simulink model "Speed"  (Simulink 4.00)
settings: Solver=ode45  StartTime=0.0  StopTime=1  MaxStep=0.0002  RelTol=1e-3
undefined symbols (not defined in the file or in its folder): const, J, No, Tf, Tmax, Ttc
libraries: simulink3 x2

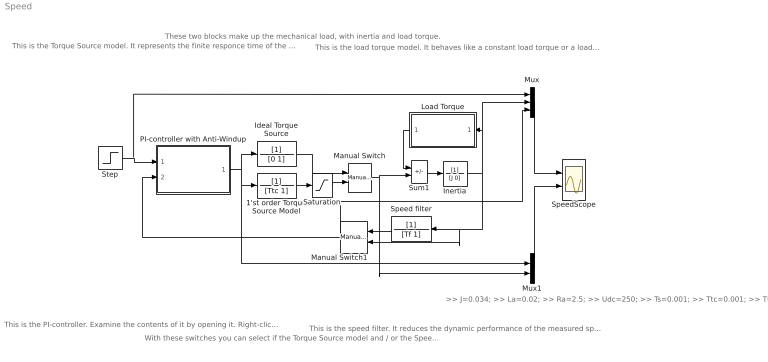
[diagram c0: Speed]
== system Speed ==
  note: This is the PI-controller. Examine the contents of it by opening it. Right-clic and select "Look under mask".
  note: With these switches you can select if the Torque Source model and / or the Speed Filter should be engaged.
  note: This is the load torque model. It behaves like a constant load torque or a load torque that is liearly or quadratically proportional to speed according to the user selection.
  note: These two blocks make up the mechanical load, with inertia and load torque.
  note: This is the Torque Source model. It represents the finite responce time of the torque loop as a 1'st order time constant and a limitation.
  note: This is the speed filter. It reduces the dynamic performance of the measured speed signal
  note: >> J=0.034; >> La=0.02; >> Ra=2.5; >> Udc=250; >> Ts=0.001; >> Ttc=0.001; >> Tf=0.05; >> Tmax=round(10*(16+rand*4))/10;
  1'st order Torque Source Model : TransferFcn  Numerator=[1]  Denominator=[Ttc 1]  AbsoluteTolerance=auto  Realization=auto
  Ideal Torque Source : TransferFcn  Numerator=[1]  Denominator=[0 1]  AbsoluteTolerance=auto  Realization=auto
  Inertia : TransferFcn  Numerator=[1]  Denominator=[J 0]  AbsoluteTolerance=auto  Realization=auto
  Load Torque : Subsystem  Orientation=left  mask(Speed dependent load){type=const, wn=100, Tn=0}
      mask prompts: type "Load type"; wn "Nominal speed [rad/s]"; Tn "Nominal load torque [Nm]"
      mask help: Either constant load torque, linearly dependent of speed or quadratically dependent of speed.
  Manual Switch : simulink3/Nonlinear/Manual Switch  sw=1  action=0
  Manual Switch1 : simulink3/Nonlinear/Manual Switch  Orientation=left  sw=0  action=0
  Mux : Mux  Inputs=3
  Mux1 : Mux  Inputs=2
  PI-controller with Anti-Windup : Subsystem  mask{Kp=0, Ti=inf, Ttc=Ttc, Limitoutput=No, Out_max=Tmax, Out_min=-Tmax}
      mask prompts: Kp "Gain"; Ti "Integral time constant"; Ttc "Controller Sampling Time"; Limitoutput "Limit the output"; Out_max "Max Controller Output (if limited)     INCLUDES Anti Windup !!"; Out_min "Min Controller Output (if limited)     INCLUDES Anti Windup !!"
  Saturation : Saturate  UpperLimit=Tmax  LowerLimit=-Tmax  LinearizeAsGain=on
  Speed filter : TransferFcn  Orientation=left  Numerator=[1]  Denominator=[Tf 1]  AbsoluteTolerance=auto  Realization=auto
  SpeedScope : Scope  NumInputPorts=2
  Step : Step  Time=0.2  Before=0  After=100  SampleTime=0
  Sum1 : Sum  Inputs=-+  SaturateOnIntegerOverflow=on
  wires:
  Inertia/1 -> Speed filter/1, Manual Switch1/2, Load Torque/1(w), Mux/2
  Mux/1 -> SpeedScope/1
  Sum1/1 -> Inertia/1
  Load Torque/1(Tl) -> Sum1/1
  Mux1/1 -> SpeedScope/2
  Step/1 -> PI-controller with Anti-Windup/1(Ref), Mux/1
  PI-controller with Anti-Windup/1(Out) -> 1'st order Torque Source Model/1, Mux1/1, Ideal Torque Source/1
  1'st order Torque Source Model/1 -> Saturation/1
  Manual Switch/1 -> Sum1/2, Mux1/2
  Speed filter/1 -> Manual Switch1/1
  Manual Switch1/1 -> PI-controller with Anti-Windup/2(Act), Mux/3
  Saturation/1 -> Manual Switch/2
  Ideal Torque Source/1 -> Manual Switch/1

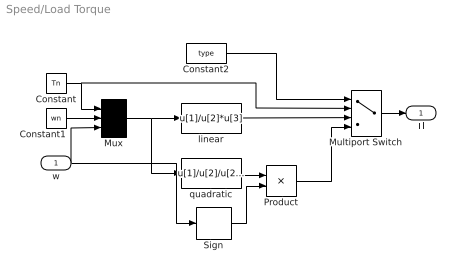
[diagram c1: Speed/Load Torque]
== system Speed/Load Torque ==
  w : Inport  Port=1  LatchInput=off
  Constant : Constant  Value=Tn
  Constant1 : Constant  Value=wn
  Constant2 : Constant  Value=type
  Multiport Switch : MultiPortSwitch  Inputs=3
  Mux : Mux  Inputs=3
  Product : Product  Inputs=2  Multiplication=Element-wise(.*)  SaturateOnIntegerOverflow=on
  Sign : Signum
  linear : Fcn  Expr=u[1]/u[2]*u[3]
  quadratic : Fcn  Expr=u[1]/u[2]/u[2]*u[3]*u[3]
  Tl : Outport  Port=1  InitialOutput=0
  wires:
  Product/1 -> Multiport Switch/4
  Multiport Switch/1 -> Tl/1
  Sign/1 -> Product/2
  quadratic/1 -> Product/1
  w/1 -> Sign/1, Mux/3
  Constant2/1 -> Multiport Switch/1
  linear/1 -> Multiport Switch/3
  Constant/1 -> Multiport Switch/2, Mux/1
  Mux/1 -> quadratic/1, linear/1
  Constant1/1 -> Mux/2

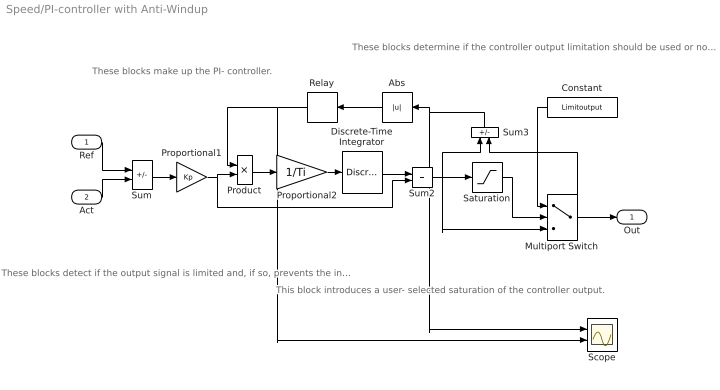
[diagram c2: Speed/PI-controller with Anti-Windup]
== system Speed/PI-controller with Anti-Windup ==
  note: These blocks make up the PI- controller.
  note: These blocks detect if the output signal is limited and, if so, prevents the integrator from integrating.
  note: This block introduces a user- selected saturation of the controller output.
  note: These blocks determine if the controller output limitation should be used or not.
  Ref : Inport  Port=1  LatchInput=off
  Act : Inport  Port=2  LatchInput=off
  Abs : Abs  Orientation=left  SaturateOnIntegerOverflow=on
  Constant : Constant  Orientation=left  Value=Limitoutput
  Discrete-Time Integrator : DiscreteIntegrator  IntegratorMethod=ForwardEuler  ExternalReset=none  InitialConditionSource=internal  InitialCondition=0  LimitOutput=off  UpperSaturationLimit=inf  LowerSaturationLimit=-inf  ShowSaturationPort=off  ShowStatePort=off  SampleTime=Ttc
  Multiport Switch : MultiPortSwitch  Inputs=2
  Product : Product  Inputs=2  Multiplication=Element-wise(.*)  SaturateOnIntegerOverflow=on
  Proportional1 : Gain  Gain=Kp  Multiplication=Element-wise(K.*u)  SaturateOnIntegerOverflow=on
  Proportional2 : Gain  Gain=1/Ti  Multiplication=Element-wise(K.*u)  SaturateOnIntegerOverflow=on
  Relay : Relay  Orientation=left  OnSwitchValue=eps  OffSwitchValue=eps  OnOutputValue=0  OffOutputValue=1
  Saturation : Saturate  UpperLimit=Out_max  LowerLimit=Out_min  LinearizeAsGain=on
  Scope : Scope  NumInputPorts=2
  Sum : Sum  Inputs=+-  SaturateOnIntegerOverflow=on
  Sum2 : Sum  Inputs=++  SaturateOnIntegerOverflow=on
  Sum3 : Sum  Orientation=up  Inputs=+-  SaturateOnIntegerOverflow=on
  Out : Outport  Port=1
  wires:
  Sum/1 -> Proportional1/1
  Discrete-Time Integrator/1 -> Sum2/1
  Proportional1/1 -> Product/2, Sum2/2
  Proportional2/1 -> Discrete-Time Integrator/1
  Sum2/1 -> Saturation/1, Sum3/1, Multiport Switch/3
  Product/1 -> Proportional2/1
  Sum3/1 -> Abs/1, Scope/1
  Abs/1 -> Relay/1
  Relay/1 -> Product/1, Scope/2
  Ref/1 -> Sum/1
  Act/1 -> Sum/2
  Saturation/1 -> Multiport Switch/2
  Constant/1 -> Multiport Switch/1
  Multiport Switch/1 -> Sum3/2, Out/1
